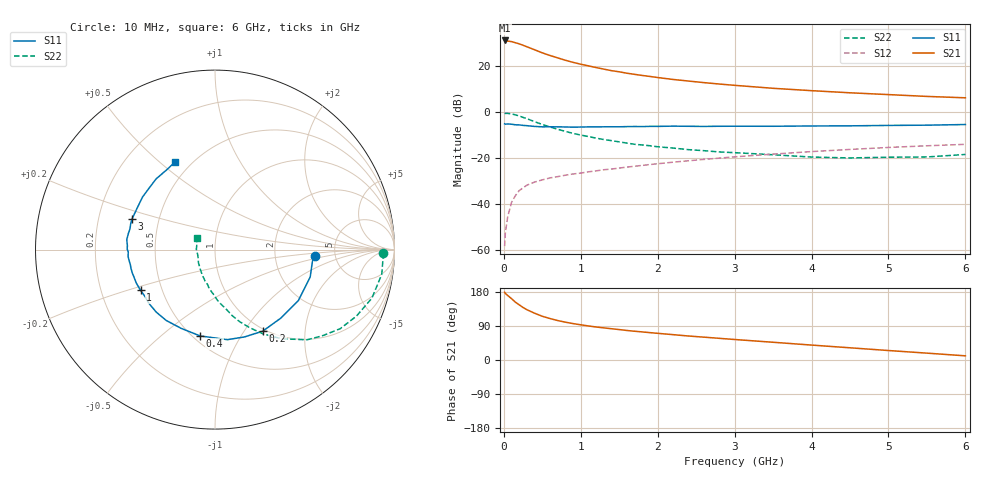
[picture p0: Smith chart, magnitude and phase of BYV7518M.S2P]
! SIEMENS Small Signal Semiconductors
! BFY420
! Si NPN RF SIEGET Grounded Emitter Transistor in MICRO-X
! VCE = 0.75 V  IC = 18 mA
! Common Emitter S-Parameters:  October  1996
# GHz  S  MA  R  50
!  f  S11  S21  S12  S22
! GHz  MAG  ANG  MAG  ANG  MAG  ANG  MAG  ANG
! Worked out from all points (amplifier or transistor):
!   36 points, 10 MHz to 6 GHz, reference 50 ohm
!   highest |S21| = 31.2 dB at 10 MHz (marker M1)
!   |S21| within 3 dB of that: start of sweep to 318.7 MHz
!   unconditionally stable (mu >= 1): 1.776 GHz to end of sweep
!   at 250 MHz: K = 0.29, MSG = 31.1 dB, |S12| = -33.0 dB
!   at 1.4 GHz: K = 0.93, MSG = 21.4 dB, |S12| = -24.8 dB
!   at 6 GHz: K = 1.10, MAG = 8.2 dB, |S12| = -14.0 dB
!   S11 on the Smith chart (normalised r, x): 10 MHz: 3.46, -0.38; 200 MHz: 0.97, -1.22; 400 MHz: 0.54, -0.69; 1 GHz: 0.38, -0.22; 3 GHz: 0.35, +0.16; 6 GHz: 0.41, +0.56
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0.01  0.5564 -3.9  36.41 178.8  0.0012 101.0  0.9388 -1.2
0.02  0.5468 -6.7  36.04 175.6  0.0024 86.3  0.9375 -2.9
0.05  0.552 -16.1  35.29 170.2  0.0052 84.6  0.9392 -8.4
0.1  0.5445 -31.5  34.38 161.9  0.0108 78.2  0.9151 -17.2
0.15  0.5294 -46.1  32.47 152.6  0.0151 72.4  0.8708 -25.2
0.2  0.5265 -59.6  30.75 145.6  0.0195 67.3  0.8249 -32.3
0.25  0.5136 -71.4  28.59 138.5  0.0224 63.2  0.7667 -38.8
0.3  0.5064 -82.2  26.51 132.7  0.0256 60.1  0.718 -44.4
0.4  0.488 -99.7  22.82 123.4  0.0299 56.1  0.6189 -53.4
0.5  0.4776 -113.3  19.55 115.4  0.0334 53.1  0.5379 -60.5
0.6  0.4793 -124.6  17.14 109.4  0.0368 51.6  0.4745 -66.2
0.7  0.478 -133.2  15.2 104.1  0.0393 50.8  0.4236 -71.2
0.8  0.4745 -141.1  13.49 99.8  0.0422 50.3  0.3803 -75.4
1  0.4727 -151.3  11.06 92.9  0.0469 50.5  0.3167 -82.1
1.1  0.4767 -157.1  10.17 89.8  0.05 51.2  0.2934 -85.8
1.6  0.4831 -173.4  7.04 77.9  0.0634 50.9  0.2115 -99.8
2.2  0.4947 173.6  5.149 66.9  0.0811 49.4  0.1648 -113.8
3  0.4928 159.7  3.834 54.1  0.106 45.5  0.1307 -130.3
3.5  0.4917 151.5  3.302 46.8  0.1216 42.2  0.1177 -141.6
4.5  0.5022 136.9  2.636 32.2  0.1537 33.6  0.1004 -164.3
5.5  0.5194 121.3  2.197 18.1  0.1846 23.8  0.1054 162.7
6  0.5366 114.5  2.05 11.0  0.1987 18.7  0.1195 148.2
